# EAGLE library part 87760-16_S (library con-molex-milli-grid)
HEADER
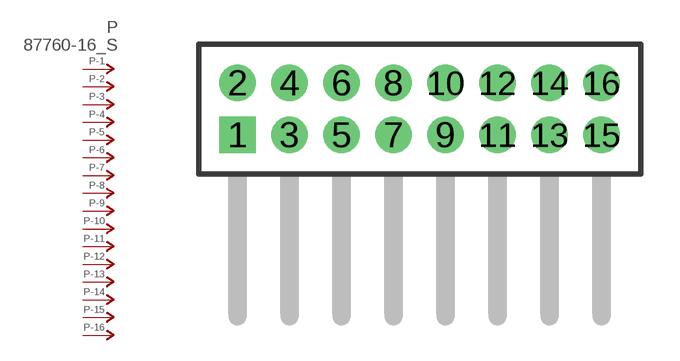
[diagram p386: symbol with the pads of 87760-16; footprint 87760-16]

Designator prefix P; gates -1=P-NV -2=P-N -3=P-N -4=P-N -5=P-N -6=P-N -7=P-N -8=P-N -9=P-N -10=P-N -11=P-N -12=P-N -13=P-N -14=P-N -15=P-N -16=P-N

## 87760-16_S  [87760-16]
1  -1:P  pas
2  -2:P  pas
3  -3:P  pas
4  -4:P  pas
5  -5:P  pas
6  -6:P  pas
7  -7:P  pas
8  -8:P  pas
9  -9:P  pas
10  -10:P  pas
11  -11:P  pas
12  -12:P  pas
13  -13:P  pas
14  -14:P  pas
15  -15:P  pas
16  -16:P  pas

## Footprint 87760-16 (pad centres in mm)
HEADER Dual Row, Right Angle
drill 0.914 square: 1 -7,-1
drill 0.914: 2 -7,1; 3 -5,-1; 4 -5,1; 5 -3,-1; 6 -3,1; 7 -1,-1; 8 -1,1; 9 1,-1; 10 1,1; 11 3,-1; 12 3,1; 13 5,-1; 14 5,1; 15 7,-1; 16 7,1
